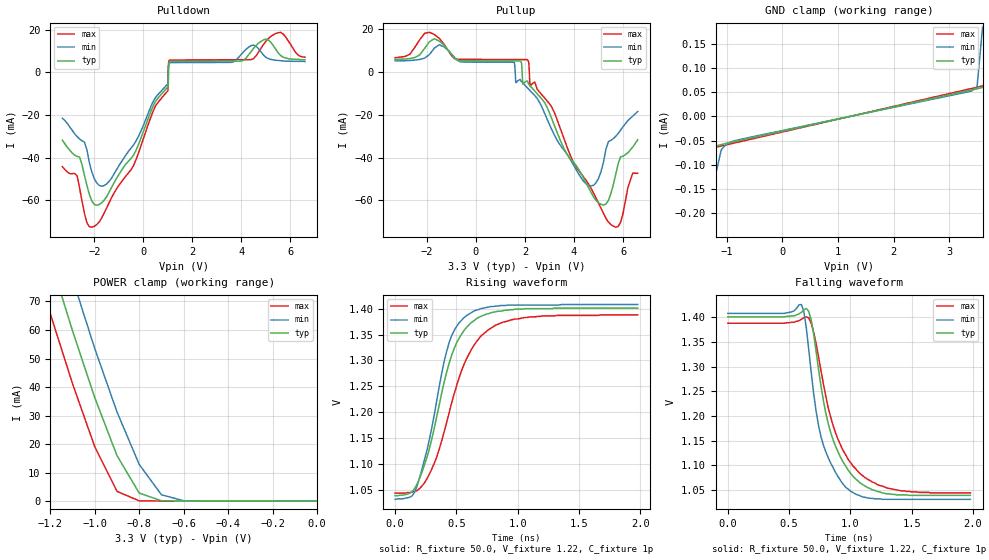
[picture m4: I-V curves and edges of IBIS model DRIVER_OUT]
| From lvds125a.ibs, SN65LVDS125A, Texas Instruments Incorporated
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|   Driver Output Model
[Model]   DRIVER_OUT
Model_type   3-state
| Signals   1Y,1Z,2Y,2Z,3Y,3Z,4Y,4Z
Vmeas = 1.22V   |Reference voltage for timing measurements
Cref = 1pF   |Timing specification test load capacitance value
Rref = 50   |Note: 50 Ohm load; single ended configuration
Vref = 1.22V   |Timing specification test load voltage
| variable   typ   min   max
C_comp   2.11pF   2.05pF   2.36pF
|   typ   min   max
[Temperature Range]   25.0   85   -40
[Voltage range]   3.3V   3.0V   3.6V
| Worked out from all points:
|   slope of the pulldown table from 0 to 0.495 V, typ, clamps not added: 34.9 ohm
|   slope of the pullup table from 0 to 0.495 V, typ, clamps not added: 25 kohm
|   GND clamp passes 1 mA (typ) near -1.61 V on its own axis
|   POWER clamp passes 1 mA (typ) near -0.73 V on its own axis
|   rising waveform, R_fixture 50.0, V_fixture 1.22, C_fixture 1p: 20-80 % time 234ps typ, 201ps min, 280ps max; typ from 1.04 V to 1.4 V
|   falling waveform, R_fixture 50.0, V_fixture 1.22, C_fixture 1p: 20-80 % time 208ps typ, 175ps min, 240ps max; typ from 1.4 V to 1.04 V
[GND_clamp]
|   Voltage   I(typ)   I(min)   I(max)
-3.6V     -101mA     -111mA     -91.7mA
-1.7V     -1.99mA    -5.02mA    -245uA
-1.6V     -887uA     -3.16mA    -91.9uA
-1.5V     -293uA     -1.77mA    -73.3uA
-1.4V     -106uA     -814uA     -69.3uA
-1.3V     -69.2uA    -305uA     -66.5uA
-1.2V     -61.5uA    -119uA     -63.9uA
-1.1V     -58.2uA    -68.9uA    -61.2uA
-1V       -55.6uA    -56.1uA    -58.6uA
3.4V      54.5uA     52.3uA     57.5uA
3.5V      57uA       59.6uA     60.2uA
3.6V      59.5uA     184uA      62.8uA
[Power_clamp]
| Note that the[POWER_clamp]voltage table is referenced to Vcc
| and is calculated using Vtable=Vcc - Vmeasured.
|   Voltage   I(typ)   I(min)   I(max)
-3.3V     812mA      831mA      791mA
-1.3V     112mA      131mA      91.8mA
-1.2V     84.9mA     104mA      65.7mA
-1.1V     59.7mA     77.9mA     41.2mA
-1V       36.3mA     53.5mA     19.1mA
-900mV    16mA       31.3mA     3.46mA
-800mV    2.86mA     12.9mA     140uA
-700mV    170uA      2.27mA     81.7uA
-600mV    69.2uA     184uA      78.6uA
0V        52uA       42.5uA     62.8uA
[Pulldown]
|   Voltage   I(typ)   I(min)   I(max)
-3.3V     -31.8mA    -21.5mA    -44.2mA
-2.7V     -39.4mA    -30.1mA    -48.5mA
-2.2V     -57.2mA    -42.3mA    -72.4mA
-1.7V     -61.2mA    -53.4mA    -68.4mA
1.01V     -6.69mA    -5.22mA    -8.49mA
1.02V     -6.56mA    -5.1mA     2.15mA
1.03V     2.6mA      2.15mA     3.84mA
1.06V     4.83mA     4.16mA     5.66mA
4.4V      9.74mA     12.6mA     5.98mA
5V        15.6mA     7.1mA      14.6mA
5.6V      8mA        5.5mA      18.8mA
6.6V      5.9mA      5.1mA      7.1mA
[Pullup]
|   Voltage   I(typ)   I(min)   I(max)
| Note that the[Pullup]voltage table is referenced to Vcc
| and is calculated using Vtable=Vcc - Vmeasured.
-3.3V     5.9mA      5.2mA      6.7mA
-1.7V     15.6mA     11.2mA     17.6mA
-800mV    5.73mA     5.96mA     5.98mA
1.56V     5.2mA      4.61mA     5.85mA
1.63V     5.2mA      -4.97mA    5.85mA
2.1V      -4.14mA    -7.41mA    5.82mA
2.21V     -6.47mA    -8.74mA    -6.44mA
3.1V      -22.1mA    -27.1mA    -16.5mA
4.6V      -54.2mA    -53.1mA    -52.5mA
5.3V      -61.8mA    -36.3mA    -68.4mA
5.7V      -48.1mA    -30.1mA    -72.6mA
6.6V      -31.7mA    -18.5mA    -47.4mA
[Ramp]
|   typ   min   max
dV/dt_r   0.200/208ps   0.200/175ps   0.200/270ps
dV/dt_f   0.200/153ps   0.200/123ps   0.200/220ps
R_load = 50ohm | Note: The measurement is on a differential configuration
|   with 100ohm line-to-line and 1p
[Rising Waveform]
R_fixture = 50.0
V_fixture = 1.22
C_fixture = 1p
L_fixture = 0n
|   V(typ)   V(min)   V(max)
0s        1.039V     1.032V     1.044V
160ps     1.053V     1.046V     1.047V
260ps     1.113V     1.127V     1.072V
340ps     1.192V     1.223V     1.114V
440ps     1.294V     1.334V     1.198V
500ps     1.333V     1.365V     1.25V
580ps     1.363V     1.386V     1.302V
700ps     1.385V     1.4V       1.347V
940ps     1.398V     1.407V     1.378V
1.98ns    1.401V     1.408V     1.388V
[Falling Waveform]
R_fixture = 50.0
V_fixture = 1.22
C_fixture = 1p
L_fixture = 0n
|   V(typ)   V(min)   V(max)
0s        1.401V     1.408V     1.388V
460ps     1.401V     1.408V     1.388V
600ps     1.41V      1.426V     1.396V
640ps     1.418V     1.379V     1.401V
680ps     1.395V     1.289V     1.388V
760ps     1.261V     1.158V     1.292V
860ps     1.151V     1.095V     1.18V
1ns       1.084V     1.048V     1.106V
1.3ns     1.042V     1.031V     1.054V
1.98ns    1.039V     1.031V     1.044V
